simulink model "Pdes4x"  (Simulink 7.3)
settings: Solver=ode45  StartTime=0.0  StopTime=50  RelTol=1e-3
undefined symbols (not defined in the file or in its folder): Aps, Bps, Cps, Dps, Kmix

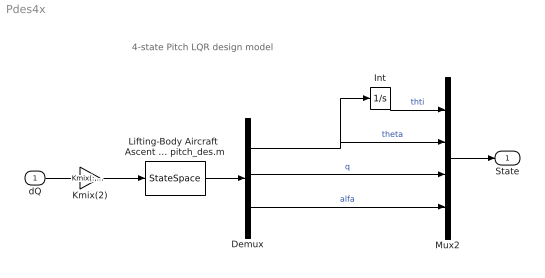
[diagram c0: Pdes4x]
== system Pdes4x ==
  note: 4-state Pitch LQR design model
  dQ : Inport  OutDataType=sfix(16)  OutScaling=2^0
  Demux : Demux  Outputs=3
  Int : Integrator
  Kmix(2) : Gain  Gain=Kmix(:,2)  ParameterDataType=sfix(16)  ParameterScaling=2^0  OutDataType=sfix(16)  OutScaling=2^0
  Lifting-Body Aircraft  Ascent Pitch Design Model from file pitch_des.m : StateSpace  A=Aps  B=Bps  C=Cps  D=Dps
  Mux2 : Mux
  State : Outport  OutDataType=sfix(16)  OutScaling=2^0
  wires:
  Lifting-Body Aircraft  Ascent Pitch Design Model from file pitch_des.m/1 -> Demux/1
  Demux/2 -> Mux2/3  "q"
  dQ/1 -> Kmix(2)/1
  Demux/3 -> Mux2/4  "alfa"
  Demux/1 -> Mux2/2, Int/1  "theta"
  Kmix(2)/1 -> Lifting-Body Aircraft  Ascent Pitch Design Model from file pitch_des.m/1
  Int/1 -> Mux2/1  "thti"
  Mux2/1 -> State/1
